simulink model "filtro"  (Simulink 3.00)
settings: Solver=ode45  StartTime=0.0  StopTime=100  MaxStep=0.1  RelTol=1e-3  AbsTol=1e-3
undefined symbols (not defined in the file or in its folder): sfunyst

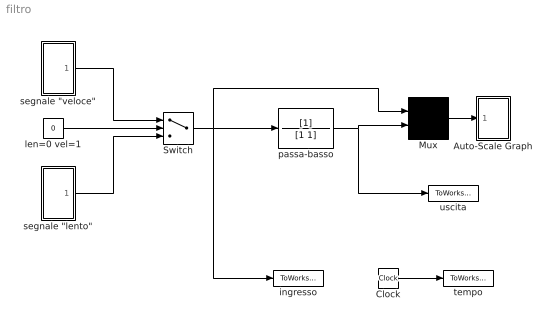
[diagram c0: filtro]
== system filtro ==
  Auto-Scale Graph : Subsystem  mask(Storage scope.){}
      mask help: Storage scope using MATLAB graph window. Enter plotting ranges and line type.
      mask init:
      | npts = @4; color = @5; ax = [0, @1, @2, @3]; dt=-1;
  Clock : Clock
  Mux : Mux  Inputs=2
  Switch : Switch  Threshold=1
  ingresso : ToWorkspace  VariableName=u  SampleTime=0  SaveFormat=Matrix
  len=0 vel=1 : Constant  Value=0
  passa-basso : TransferFcn  Numerator=[1]  Denominator=[1 1]
  "segnale \"lento\"" : Subsystem
  "segnale \"veloce\"" : Subsystem
  tempo : ToWorkspace  VariableName=t  SampleTime=0  SaveFormat=Matrix
  uscita : ToWorkspace  VariableName=yf  SampleTime=0  SaveFormat=Matrix
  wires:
  Mux/1 -> Auto-Scale Graph/1(x)
  Clock/1 -> tempo/1
  passa-basso/1 -> Mux/2, uscita/1
  len=0 vel=1/1 -> Switch/2
  "segnale \"veloce\""/1(out_1) -> Switch/1
  "segnale \"lento\""/1(out_1) -> Switch/3
  Switch/1 -> passa-basso/1, Mux/1, ingresso/1

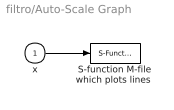
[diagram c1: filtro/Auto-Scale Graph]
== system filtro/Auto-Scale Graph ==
  x : Inport  Port=1  PortWidth=-1  SampleTime=-1  DataType=auto
  "S-function M-file which plots lines " : S-Function  LoadFcn=sfunyst([],[],[],'LoadBlock')  FunctionName=sfunyst  Parameters=ax, color, npts, dt  PortCounts=[]  SFunctionModules=''
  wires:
  x/1 -> "S-function M-file which plots lines "/1

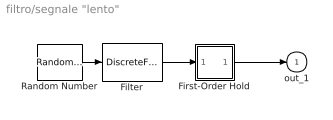
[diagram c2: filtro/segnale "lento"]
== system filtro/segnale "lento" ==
  Filter : DiscreteFilter  Numerator=[1]  Denominator=[1 -0.9]  SampleTime=1
  First-Order Hold : Subsystem  mask(First-Order Hold){}
      mask help: First-Order Hold
      mask init:
      | Ts=@1;
  Random Number : RandomNumber  Mean=0  Variance=1  Seed=0  SampleTime=1
  out_1 : Outport  Port=1
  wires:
  Random Number/1 -> Filter/1
  Filter/1 -> First-Order Hold/1(input)
  First-Order Hold/1(output) -> out_1/1

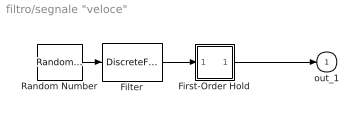
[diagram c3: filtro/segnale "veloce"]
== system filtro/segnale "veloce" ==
  Filter : DiscreteFilter  Numerator=[1]  Denominator=[1 0.9]  SampleTime=1
  First-Order Hold : Subsystem  mask(First-Order Hold){}
      mask help: First-Order Hold
      mask init:
      | Ts=@1;
  Random Number : RandomNumber  Mean=0  Variance=1  Seed=0  SampleTime=1
  out_1 : Outport  Port=1
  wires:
  Random Number/1 -> Filter/1
  Filter/1 -> First-Order Hold/1(input)
  First-Order Hold/1(output) -> out_1/1

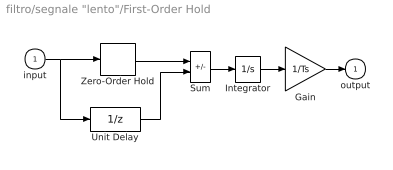
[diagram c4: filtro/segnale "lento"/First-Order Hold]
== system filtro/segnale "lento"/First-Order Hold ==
  input : Inport  Port=1  PortWidth=-1  SampleTime=-1  DataType=auto
  Gain : Gain  Gain=1/Ts  SaturateOnIntegerOverflow=on
  Integrator : Integrator  ExternalReset=none  InitialConditionSource=internal  InitialCondition=0  LimitOutput=off  UpperSaturationLimit=inf  LowerSaturationLimit=-inf  ShowSaturationPort=off  ShowStatePort=off  AbsoluteTolerance=auto
  Sum : Sum  Inputs=+-  SaturateOnIntegerOverflow=on
  Unit Delay : UnitDelay  X0=0  SampleTime=Ts
  Zero-Order Hold : ZeroOrderHold  SampleTime=Ts
  output : Outport  Port=1
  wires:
  input/1 -> Zero-Order Hold/1, Unit Delay/1
  Zero-Order Hold/1 -> Sum/1
  Unit Delay/1 -> Sum/2
  Sum/1 -> Integrator/1
  Integrator/1 -> Gain/1
  Gain/1 -> output/1

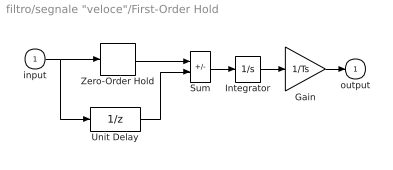
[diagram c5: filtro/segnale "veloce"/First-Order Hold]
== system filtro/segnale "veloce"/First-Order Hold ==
  input : Inport  Port=1  PortWidth=-1  SampleTime=-1  DataType=auto
  Gain : Gain  Gain=1/Ts  SaturateOnIntegerOverflow=on
  Integrator : Integrator  ExternalReset=none  InitialConditionSource=internal  InitialCondition=0  LimitOutput=off  UpperSaturationLimit=inf  LowerSaturationLimit=-inf  ShowSaturationPort=off  ShowStatePort=off  AbsoluteTolerance=auto
  Sum : Sum  Inputs=+-  SaturateOnIntegerOverflow=on
  Unit Delay : UnitDelay  X0=0  SampleTime=Ts
  Zero-Order Hold : ZeroOrderHold  SampleTime=Ts
  output : Outport  Port=1
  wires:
  input/1 -> Zero-Order Hold/1, Unit Delay/1
  Zero-Order Hold/1 -> Sum/1
  Unit Delay/1 -> Sum/2
  Sum/1 -> Integrator/1
  Integrator/1 -> Gain/1
  Gain/1 -> output/1
